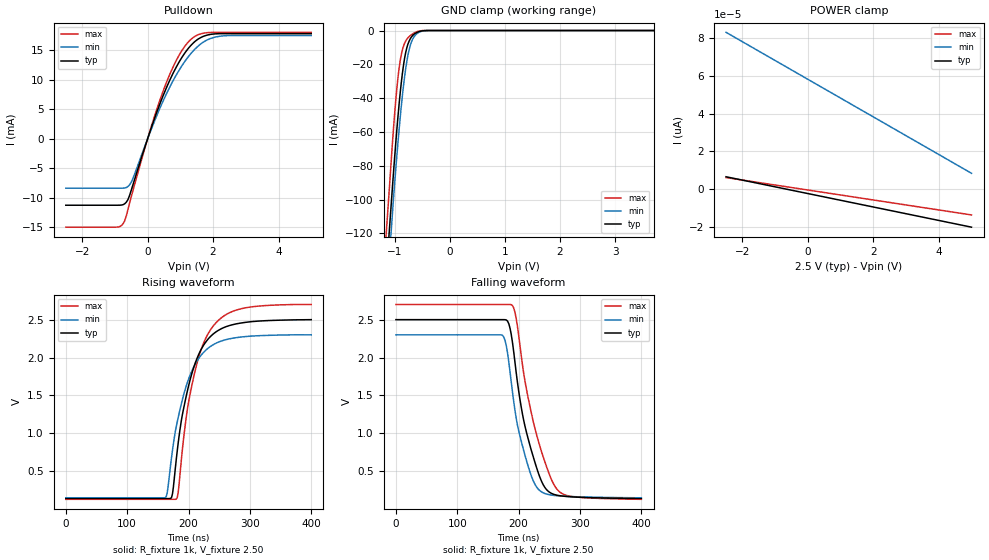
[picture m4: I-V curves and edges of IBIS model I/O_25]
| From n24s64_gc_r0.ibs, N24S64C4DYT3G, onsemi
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|//////////////////////////////////////////////////////////////////////////////
|//////////////////////////////////////////////////////////////////////////////
[Model] I/O_25
Model_type I/O_open_drain
Vinh =  1.75
Vinl =  0.75
Vmeas = 1.25
Vref = 2.50
Rref = 1000
Cref = 100pF
|  variable   typ   min   max
C_comp   8.00pF   8.00pF   8.00pF
|//////////////////////////////////////////////////////////////////////////////
[Temperature Range]   25   85   -40
|//////////////////////////////////////////////////////////////////////////////
[Voltage Range]   2.50V   2.30V   2.70V
|//////////////////////////////////////////////////////////////////////////////
[Pulldown Reference]   0V   0V   0V
|//////////////////////////////////////////////////////////////////////////////
[POWER Clamp Reference] 2.50V   2.30V   2.70V
|////////////////////////////////////////////////////////////////////////
[GND Clamp Reference]   0V   0V   0V
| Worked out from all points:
|   slope of the pulldown table from 0 to 0.375 V, typ, clamps not added: 63.3 ohm
|   GND clamp passes 1 mA (typ) near -0.59 V on its own axis
|   falling waveform, R_fixture 1k, V_fixture 2.50: 20-80 % time 34.1ns typ, 29.9ns min, 40.2ns max; typ from 2.5 V to 0.14 V
|   rising waveform, R_fixture 1k, V_fixture 2.50: 20-80 % time 36.4ns typ, 37.4ns min, 36.1ns max; typ from 0.14 V to 2.5 V
|//////////////////////////////////////////////////////////////////////////////
[Pulldown]
|   Voltage   I(typ)   I(min)   I(max)
-2.5V     -11.27mA   -8.381mA   -14.99mA
-950mV    -11.27mA   -8.381mA   -14.99mA
-750mV    -11.18mA   -8.371mA   -14.42mA
-600mV    -10.31mA   -8.088mA   -11.96mA
-500mV    -8.727mA   -7.371mA   -9.84mA
100mV     1.677mA    1.445mA    1.848mA
500mV     7.675mA    6.74mA     8.479mA
950mV     12.92mA    11.54mA    14.07mA
1.35V     16.02mA    14.65mA    17.01mA
1.75V     17.49mA    16.58mA    17.97mA
2.2V      17.85mA    17.41mA    18.08mA
5V        17.85mA    17.55mA    18.08mA
|//////////////////////////////////////////////////////////////////////////////
[GND Clamp]
|   Voltage   I(typ)   I(min)   I(max)
-2.5V     -758.6mA   -779.6mA   -739.3mA
-1.15V    -142.6mA   -158.6mA   -118.3mA
-1.12V    -128.9mA   -144.8mA   -104.5mA
-1.08V    -110.6mA   -126.4mA   -85.38mA
-1.06V    -101.5mA   -117.2mA   -75.66mA
-1V       -74.76mA   -90.26mA   -49.05mA
-940mV    -50.81mA   -66.17mA   -27.82mA
-900mV    -37mA      -51.59mA   -17.9mA
-840mV    -20.6mA    -32.69mA   -9.228mA
-740mV    -6.417mA   -11.65mA   -3.684mA
-620mV    -1.543mA   -2.556mA   -1.02mA
5V        6.52pA     85.03pA    5.573pA
|//////////////////////////////////////////////////////////////////////////////
[POWER Clamp]
|   Voltage   I(typ)   I(min)   I(max)
-2.5V     6.52pA     83.04pA    6.101pA
0V        -2.379pA   58.15pA    -498.6fA
2.5V      -11.28pA   33.26pA    -7.098pA
5V        -20.18pA   8.364pA    -13.7pA
|//////////////////////////////////////////////////////////////////////////////
|//////////////////////////////////////////////////////////////////////////////
[Ramp]
|  variable   typ   min   max
dV/dt_r   1.416E+00/3.600E-08  1.290E+00/3.750E-08  1.542E+00/3.600E-08
dV/dt_f   1.416E+00/3.400E-08  1.290E+00/3.000E-08  1.542E+00/4.000E-08
R_load = 1k
|//////////////////////////////////////////////////////////////////////////////
|//////////////////////////////////////////////////////////////////////////////
[Falling Waveform]
R_fixture = 1k
V_fixture = 2.50
V_fixture_min = 2.30
V_fixture_max = 2.70
C_fixture = 0p
|   time   V(typ)   V(min)   V(max)
0s        2.5V       2.3V       2.7V
174ns     2.5V       2.291V     2.7V
180ns     2.495V     2.151V     2.7V
190ns     2.198V     1.544V     2.685V
196ns     1.803V     1.201V     2.517V
204ns     1.357V     905.5mV    2.041V
220ns     795.5mV    454.3mV    1.296V
240ns     323.6mV    216mV      691.7mV
260ns     189.1mV    179.7mV    291.2mV
400ns     140mV      150mV      130mV
|//////////////////////////////////////////////////////////////////////////////
[Rising Waveform]
R_fixture = 1k
V_fixture = 2.50
V_fixture_min = 2.30
V_fixture_max = 2.70
C_fixture = 0p
|   time   V(typ)   V(min)   V(max)
0s        140mV      150mV      130mV
162ns     140mV      151.4mV    130mV
172.5ns   157.2mV    692.7mV    130mV
180ns     652.8mV    1.089V     132.6mV
189ns     1.202V     1.413V     706.4mV
205.5ns   1.791V     1.824V     1.634V
220.5ns   2.106V     2.03V      2.104V
237ns     2.287V     2.153V     2.38V
285ns     2.455V     2.27V      2.643V
400ns     2.5V       2.3V       2.7V
